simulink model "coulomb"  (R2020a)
settings: Solver=ode45  StartTime=0.0  StopTime=10.0  MaxStep=0.01  RelTol=1e-3  EnableMultiTasking=on

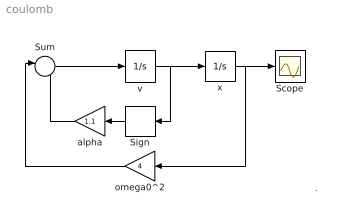
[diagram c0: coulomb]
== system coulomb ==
  note: .
  Scope : Scope
  Sign : Signum
  Sum : Sum  Inputs=|--  InputSameDT=on  SaturateOnIntegerOverflow=on
  alpha : Gain  Gain=1.1  SaturateOnIntegerOverflow=on
  omega0^2 : Gain  Gain=4  SaturateOnIntegerOverflow=on
  v : Integrator
  x : Integrator  InitialCondition=3
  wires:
  v/1 -> x/1, Sign/1
  x/1 -> omega0^2/1, Scope/1
  Sum/1 -> v/1
  Sign/1 -> alpha/1
  alpha/1 -> Sum/2
  omega0^2/1 -> Sum/1
